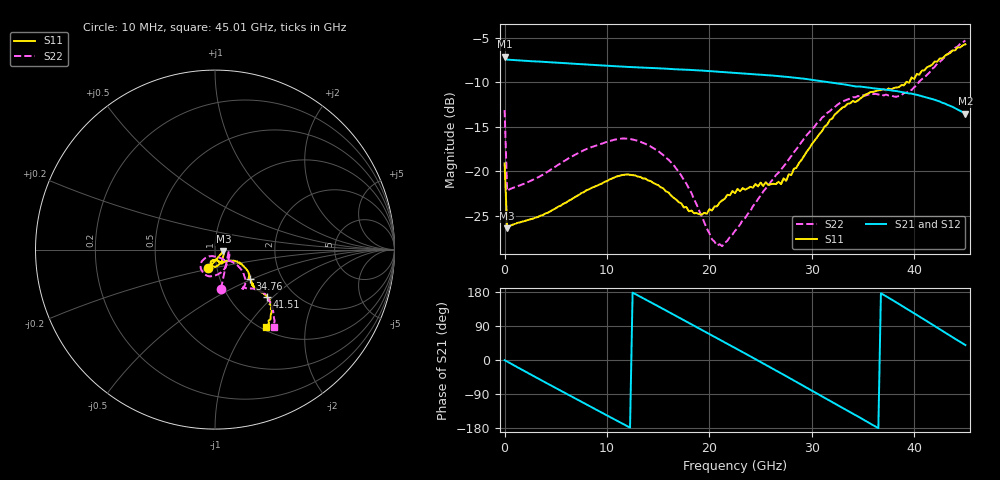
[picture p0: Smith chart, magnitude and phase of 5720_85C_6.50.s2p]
! Device:  ADRF5720
! Description: 0.5dB LSB GaAs MMIC 6-bit Digital Attenuator
! Frequency:  0.000009 -  40 GHz
! Ports:
!	RF1	= Port 1
!	RF2	= Port 2
! Vdd:  3.3 Volt
! Vss:  -3.3 Volt
! Control:  0/3.3 Volt
! State:  6.50 dB attenuation
! Data:  The device was measured using G-S-G Probes on a matrix board.
!  Data was collected using an calibrated 4 port network analyzer.
!  The reference plane for this measurement is at the launchers.
! Note:  Analog Devices supplies this data as a sample of measured data
!  for this product.  Your particular data for this product may vary.
!  Data was taken at 85 degrees C.
!  Analog Devices reserves the right to change this data at anytime.
# GHZ S DB R 45.0
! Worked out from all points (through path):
!   181 points, 10 MHz to 45.01 GHz, reference 45 ohm
!   highest |S21| = -7.15 dB at 10 MHz (marker M1); lowest = -13.5 dB at 45.01 GHz (marker M2)
!   group delay of S21, straight-line fit = 41.5 ps
!   lowest |S11| = -26.4 dB at 260 MHz (marker M3), VSWR 1.10, Z = 49.4 - j0.834 ohm
!   |S11| at or under -10 dB: start of sweep to 39.23 GHz; 39.34929 GHz to 39.54629 GHz (197 MHz wide, 0.499 % of centre)
!   |S22| runs from -28.4 to -5.3 dB; largest |S21 - S12| = 0.0022
!   S11 on the Smith chart (normalised r, x): 10 MHz: 0.91, -0.19; 34.76 GHz: 1.38, -0.49; 41.51 GHz: 1.47, -0.91; 45.01 GHz: 1.06, -1.24
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0.01  -19.12 -109.1  -7.15 -0.6  -7.14 -0.6  -13.14 -81.3
0.26  -26.40 -10.1  -7.47 -4.0  -7.46 -4.0  -22.22 -7.1
2.01  -25.57 -16.7  -7.60 -30.2  -7.59 -30.2  -21.37 -19.5
4.26  -24.65 -39.5  -7.75 -63.1  -7.74 -63.1  -20.03 -45.3
6.01  -23.53 -51.1  -7.87 -88.5  -7.86 -88.5  -18.74 -60.9
7.76  -22.35 -61.5  -8.00 -113.8  -7.98 -113.8  -17.64 -74.4
11.51  -20.43 -87.4  -8.26 -167.8  -8.24 -167.7  -16.33 -103.2
13.26  -20.64 -98.5  -8.36 167.1  -8.34 167.2  -16.69 -115.8
15.26  -21.81 -107.3  -8.46 138.1  -8.44 138.2  -17.98 -129.3
18.01  -24.51 -101.1  -8.62 98.1  -8.61 98.3  -21.95 -139.0
20.76  -23.95 -75.8  -8.81 57.7  -8.80 57.9  -28.36 -108.2
22.76  -21.98 -67.9  -8.97 28.2  -8.95 28.4  -26.37 -66.2
24.51  -21.44 -65.5  -9.12 2.3  -9.10 2.5  -23.57 -52.4
26.26  -21.42 -55.9  -9.27 -23.9  -9.25 -23.6  -20.86 -42.0
27.51  -21.08 -44.4  -9.40 -42.7  -9.39 -42.4  -19.09 -35.5
30.26  -16.60 -29.7  -9.78 -84.5  -9.76 -84.2  -15.03 -36.7
32.26  -13.64 -32.2  -10.09 -114.9  -10.07 -114.6  -12.79 -43.4
34.76  -11.84 -40.3  -10.50 -152.8  -10.49 -152.5  -11.61 -53.1
37.76  -10.84 -43.0  -10.93 160.1  -10.91 160.5  -11.49 -54.1
39.76  -9.47 -43.2  -11.29 127.3  -11.27 127.7  -10.88 -49.4
41.51  -8.21 -42.4  -11.83 98.0  -11.80 98.4  -8.91 -41.6
45.01  -5.75 -56.3  -13.53 39.4  -13.49 39.8  -5.32 -52.8
